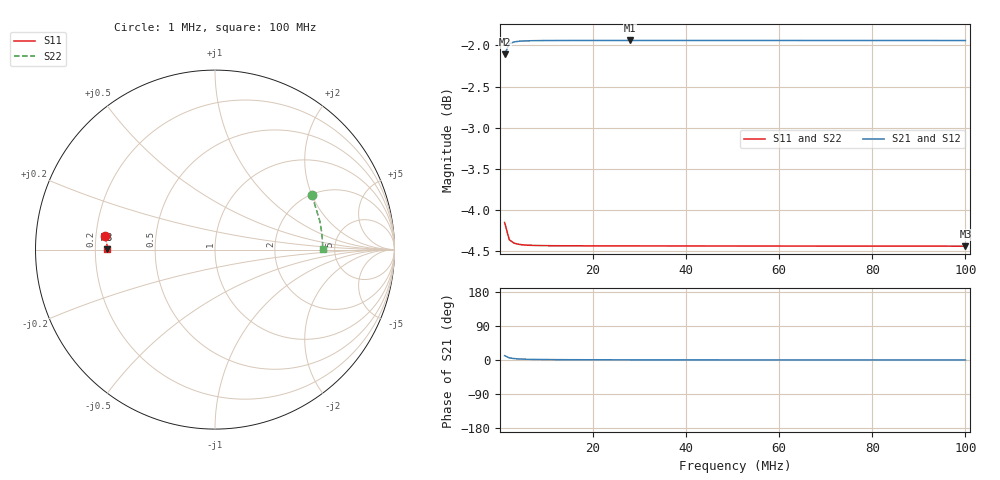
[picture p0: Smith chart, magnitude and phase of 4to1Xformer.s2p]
# MHz S RI R 50.0
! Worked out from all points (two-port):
!   100 points, 1 MHz to 100 MHz, reference 50 ohm
!   highest |S21| = -1.94 dB at 28 MHz (marker M1); lowest = -2.1 dB at 1 MHz (marker M2)
!   |S21| within 3 dB of the highest: start of sweep to end of sweep
!   lowest |S11| = -4.4 dB at 100 MHz (marker M3), VSWR 4.00, Z = 12.5 + j0.0311 ohm
!   |S11| at or under -10 dB: nowhere
!   |S22| runs from -4.4 to -4.2 dB; largest |S21 - S12| = 0
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1  -0.6152 0.0765  0.7695 0.1531  0.7695 0.1531  0.5391 0.3062
2  -0.6039 0.0394  0.7922 0.0788  0.7922 0.0788  0.5843 0.1576
3  -0.6017 0.0264  0.7965 0.0528  0.7965 0.0528  0.593 0.1056
4  -0.601 0.0198  0.798 0.0397  0.798 0.0397  0.5961 0.0794
5  -0.6006 0.0159  0.7987 0.0318  0.7987 0.0318  0.5975 0.0636
6  -0.6004 0.0132  0.7991 0.0265  0.7991 0.0265  0.5982 0.053
7  -0.6003 0.0114  0.7993 0.0227  0.7993 0.0227  0.5987 0.0454
8  -0.6002 0.00994  0.7995 0.0199  0.7995 0.0199  0.599 0.0398
9  -0.6002 0.00884  0.7996 0.0177  0.7996 0.0177  0.5992 0.0353
10  -0.6001 0.00796  0.7997 0.0159  0.7997 0.0159  0.5994 0.0318
11  -0.6001 0.00723  0.7997 0.0145  0.7997 0.0145  0.5995 0.0289
13  -0.6001 0.00612  0.7998 0.0122  0.7998 0.0122  0.5996 0.0245
15  -0.6 0.0053  0.7998 0.0106  0.7998 0.0106  0.5997 0.0212
18  -0.6 0.00442  0.7999 0.00884  0.7999 0.00884  0.5998 0.0177
22  -0.6 0.00362  0.7999 0.00723  0.7999 0.00723  0.5999 0.0145
28  -0.5999 0.00284  0.7999 0.00568  0.7999 0.00568  0.5999 0.0114
34  -0.5999 0.00234  0.7999 0.00468  0.7999 0.00468  0.6 0.00936
42  -0.5999 0.00189  0.7999 0.00379  0.7999 0.00379  0.6 0.00758
51  -0.5999 0.00156  0.7999 0.00312  0.7999 0.00312  0.6 0.00624
67  -0.5998 0.00119  0.7999 0.00238  0.7999 0.00238  0.6 0.00475
84  -0.5998 0.000948  0.7999 0.00189  0.7999 0.00189  0.6 0.00379
100  -0.5997 0.000796  0.7999 0.00159  0.7999 0.00159  0.6001 0.00318
